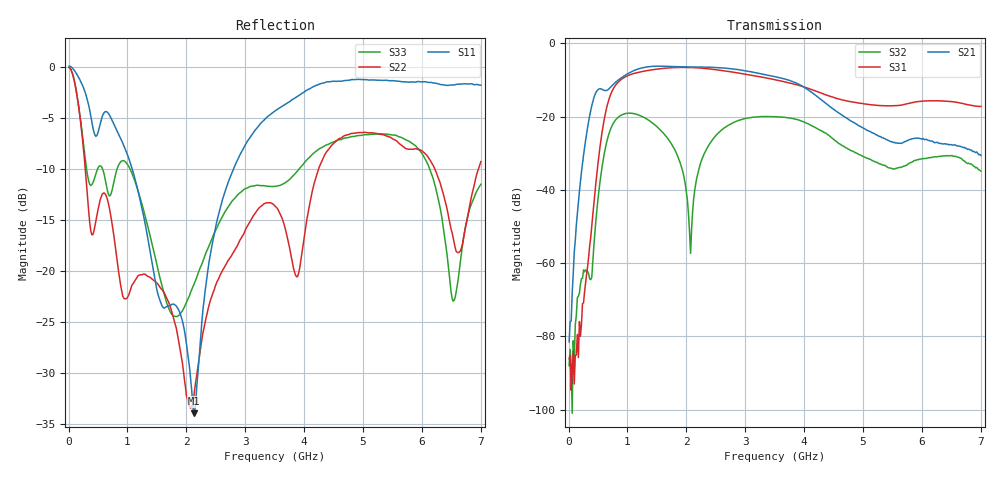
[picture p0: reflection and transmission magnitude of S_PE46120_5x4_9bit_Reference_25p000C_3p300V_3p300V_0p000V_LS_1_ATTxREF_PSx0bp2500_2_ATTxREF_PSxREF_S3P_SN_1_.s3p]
! Device ID: PE46120_5x4_9bit_Reference
! Device ID: PE46120_5x4_9bit_Reference
! File Path: z:\PE46120_5x4_9bit_Reference\MPAC_Yi\new_12port\25p000C\3p300\LS_1_ATTxREF_PSx0bp2500_2_ATTxREF_PSxREF\PE46120_5x4_9bit_Reference_25p000C_3p300V_3p300V_0p000V_LS_1_ATTxREF_PSx0bp2500_2_ATTxREF_PSxREF_S3P_SN_1_.s3p
! Serial: 1
! Lot:
! Temp: 25.000C
! VDD: 3.300
! VSS: 0.000
! Control_Hi: 3.300
! Control_Lo: 0.000
! Logic State: LS_1_ATTxREF_PSx0bp2500_2_ATTxREF_PSxREF
! Port 1: RFin
! Port 2: RFout1
! Port 3: RFout2
! ThroughPath:1-2
! IDD: -0.0005401476
! ISS: 0
! Comment:
#  Hz  S  RI  R  50
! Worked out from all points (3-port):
!   401 points, 10 MHz to 7 GHz, reference 50 ohm
!   strongest paths, dB at 10 MHz, 1.758 GHz, 3.505 GHz, 5.253 GHz, 7 GHz:
!     S21: -81.5, -6.3, -9.1, -25.1, -30.6
!     S31: -86.1, -6.6, -9.9, -16.9, -17.2
!     S32: -88.0, -27.7, -20.0, -32.6, -34.9
!   lowest |S11| = -34.0 dB at 2.124 GHz (marker M1), VSWR 1.04, Z = 50.9 + j1.81 ohm
!   |S11| at or under -10 dB: 1.08 GHz to 2.801 GHz (1.721 GHz wide, 88.7 % of centre)
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1e7  1.002 -0.1147  7.18e-05 -6.3e-05  7.48e-05 4.76e-06
     4.1e-05 -7.34e-05  0.9888 -0.0956  -2.36e-05 -7.25e-05
     -3.85e-06 4.93e-05  1.61e-05 3.64e-05  0.9882 -0.096
2.37175e8  -0.4718 -0.6617  -0.0217 -0.00712  3.51e-06 0.000273
           -0.0219 -0.00726  -0.2761 -0.3459  -0.000251 0.000514
           1.69e-05 0.00028  -0.000193 0.000591  -0.2972 -0.3509
4.6435e8  -0.4446 -0.1038  -0.0243 0.2089  0.0118 0.00325
          -0.0244 0.2119  0.1533 0.0856  -0.00247 0.00296
          0.012 0.00324  -0.00245 0.00294  0.1552 0.2562
9.71125e8  -0.2403 0.3069  0.301 -0.2102  -0.0701 0.3408
           0.3052 -0.213  -0.00774 0.0726  -0.00015 0.1093
           -0.0709 0.3455  -6.9e-05 0.1106  0.0771 -0.332
1.408e9  -0.0296 0.1101  -0.2822 -0.3879  0.4128 -0.1223
         -0.2862 -0.393  0.0653 -0.0642  -0.00312 -0.0832
         0.4175 -0.1241  -0.00333 -0.0841  -0.1346 -0.0342
2.124475e9  0.00925 0.0178  -0.1671 0.4403  -0.4069 -0.2184
            -0.169 0.4463  0.0185 -0.0149  -0.00402 -0.00642
            -0.4123 -0.2212  -0.00414 -0.00644  -0.0827 0.0207
2.77105e9  -0.00462 -0.3009  0.4435 0.0427  -0.1254 0.3834
           0.4497 0.0428  -0.0368 -0.1134  0.0185 0.0781
           -0.1265 0.3887  0.0187 0.0789  0.0458 0.2139
3.505e9  -0.4757 -0.3793  -0.1383 -0.3179  0.3115 0.0503
         -0.1405 -0.3223  0.00177 0.2079  -0.00429 -0.0988
         0.3157 0.051  -0.00436 -0.1001  0.1836 -0.1835
6.213625e9  -0.3942 0.7343  0.022 -0.0384  -0.029 0.1602
            0.0221 -0.0383  0.1621 -0.274  -0.0273 0.00502
            -0.0296 0.1628  -0.028 0.00484  0.2324 -0.1336
7e9  -0.1146 0.805  -0.0254 -0.0152  0.1236 0.0554
     -0.0254 -0.0152  -0.00926 0.3432  0.0184 -0.00195
     0.1266 0.0561  0.0179 -0.00214  0.1474 0.2214
